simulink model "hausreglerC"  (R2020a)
settings: Solver=ode45  StartTime=0.0  StopTime=400  MaxStep=1  RelTol=1e-3  EnableMultiTasking=on
undefined symbols (not defined in the file or in its folder): sigbuilder_block
libraries: libregler1B x2

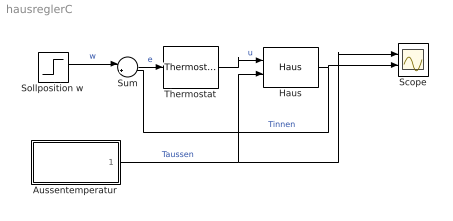
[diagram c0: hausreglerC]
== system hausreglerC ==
  Aussentemperatur : Subsystem  Tag=STV Subsys  LoadFcn=sigbuilder_block('load');  StartFcn=sigbuilder_block('start');  StopFcn=sigbuilder_block('stop');  ClipboardFcn=sigbuilder_block('clipboard');  mask(Sigbuilder block){tuvar=[0:10]}
      mask help: Create and generate interchangeable groups of signals whose waveforms are piecewise linear.
      mask init:
      | if ~strcmp(get_param(bdroot(gcbh),'SimulationStatus'),'stopped') tuvar = sigbuilder_block('maskInit'); end
  Haus : libregler1B/Haus  C=100000  R=0.001  T0=16
  Scope : Scope  NumInputPorts=2
  Sollposition w : Step  Time=300  Before=20  After=20  SampleTime=0
  Sum : Sum  Inputs=|+-  SaturateOnIntegerOverflow=on
  Thermostat : libregler1B/Thermostat  umax=18500  delta=0.5
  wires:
  Thermostat/1 -> Haus/1  "u"
  Haus/1 -> Sum/2, Scope/2  "Tinnen"
  Sollposition w/1 -> Sum/1  "w"
  Sum/1 -> Thermostat/1  "e"
  Aussentemperatur/1(Signal 1) -> Scope/1, Haus/2  "Taussen"

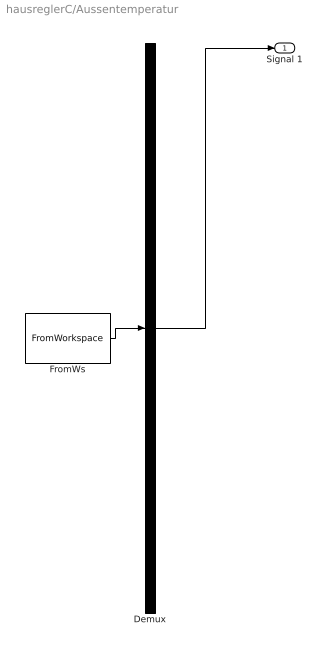
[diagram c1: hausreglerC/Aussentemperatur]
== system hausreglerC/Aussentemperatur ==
  Demux : Demux  Tag=STV Demux  Outputs=1
  FromWs : FromWorkspace  Tag=STV FromWs  VariableName=tuvar
  Signal 1 : Outport  Tag=STV Outport
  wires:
  Demux/1 -> Signal 1/1
  FromWs/1 -> Demux/1
